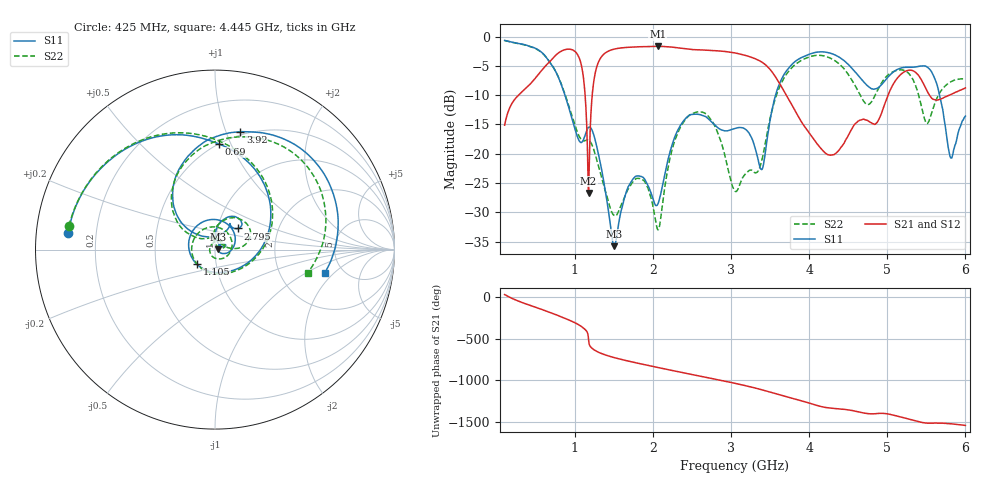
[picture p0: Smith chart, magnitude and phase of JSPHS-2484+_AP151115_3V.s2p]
!Mini-Circuits Laboratory
!S-Parameters
!Run/Lot/Date Code:MF33450/NA/1551
!Fixture/SN/Due: 90-4-20-21/70546/03/17/16
!Connection:PORT<IN> - pin<1>; PORT<OUT> - pin<7>;PORT<BIAS> - pin<4>;
!Tested With:PORT EXTENTION
!Network Analyzer:AG E5071C/74883/05/12/16
!Created: 01-07-2016 at 14:09:21
!MODEL: JSPHS-2484+
!S/N: V=3V
# MHZ S DB R 50
!Frequency  S11 dB  S11 DEG  S21 dB  S21 DEG  S12 dB  S12 DEG  S22 dB  S22 DEG
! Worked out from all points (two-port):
!   1181 points, 100 MHz to 6 GHz, reference 50 ohm
!   highest |S21| = -1.66 dB at 2.06 GHz (marker M1); lowest = -26.7 dB at 1.175 GHz (marker M2)
!   |S21| within 3 dB of the highest: 649.4 MHz to 1.079 GHz (429.3 MHz wide, 49.7 % of centre); 1.293 GHz to 3.426 GHz (2.134 GHz wide, 90.4 % of centre)
!   lowest |S11| = -35.8 dB at 1.505 GHz (marker M3), VSWR 1.03, Z = 51.6 + j0.26 ohm
!   |S11| at or under -10 dB: 872.7 MHz to 3.569 GHz (2.696 GHz wide, 121 % of centre); 5.67 GHz to end of sweep
!   |S22| runs from -33.0 to -0.7 dB; largest |S21 - S12| = 0.0024
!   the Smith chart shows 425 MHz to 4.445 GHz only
!   S11 on the Smith chart (normalised r, x): 425 MHz: 0.10, +0.05; 690 MHz: 0.50, +0.91; 1.105 GHz: 0.81, -0.13; 2.795 GHz: 1.26, +0.31; 3.92 GHz: 0.47, +1.12; 4.445 GHz: 3.66, -1.54
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100  -0.65 -58.4  -15.12 31.3  -15.11 31.2  -0.65 -58.4
425  -1.69 173.7  -8.14 -98.6  -8.13 -98.6  -1.67 170.7
690  -4.61 87.7  -4.11 172.6  -4.11 172.6  -4.57 84.2
915  -11.81 1.2  -2.13 88.0  -2.13 88.0  -11.53 0.6
1085  -18.07 -115.3  -5.01 5.3  -5.01 5.3  -17.61 -103.4
1105  -17.74 -141.4  -6.56 -8.7  -6.56 -8.7  -17.79 -127.3
1175  -15.49 118.8  -26.71 -153.6  -26.71 -153.5  -17.68 125.8
1295  -19.68 7.9  -4.57 59.9  -4.56 59.9  -21.76 -17.3
1505  -35.79 8.9  -2.12 -8.4  -2.12 -8.4  -30.53 180.0
2060  -28.64 53.3  -1.66 -126.6  -1.66 -126.6  -32.95 44.6
2070  -28.34 59.0  -1.66 -128.6  -1.66 -128.6  -32.95 54.6
2360  -14.98 72.7  -1.99 174.6  -1.99 174.6  -15.25 72.5
2795  -15.12 42.3  -2.40 93.1  -2.40 93.1  -15.37 9.4
3050  -15.68 59.9  -2.78 42.3  -2.79 42.2  -26.40 44.0
3480  -15.85 142.4  -5.31 -58.7  -5.32 -58.8  -15.14 149.0
3920  -3.46 77.9  -14.95 -173.4  -14.94 -173.2  -3.92 79.7
4035  -2.85 60.9  -17.10 153.6  -17.09 153.6  -3.33 61.3
4445  -4.07 -11.8  -18.24 89.1  -18.21 88.9  -5.46 -13.8
5020  -6.74 141.6  -9.65 31.3  -9.65 31.2  -6.44 109.1
5500  -5.10 21.7  -9.04 -76.5  -9.05 -76.5  -14.81 57.0
5810  -20.68 1.1  -9.91 -84.9  -9.91 -84.9  -7.74 72.9
6000  -13.58 33.2  -8.76 -105.0  -8.77 -105.1  -7.28 57.6
